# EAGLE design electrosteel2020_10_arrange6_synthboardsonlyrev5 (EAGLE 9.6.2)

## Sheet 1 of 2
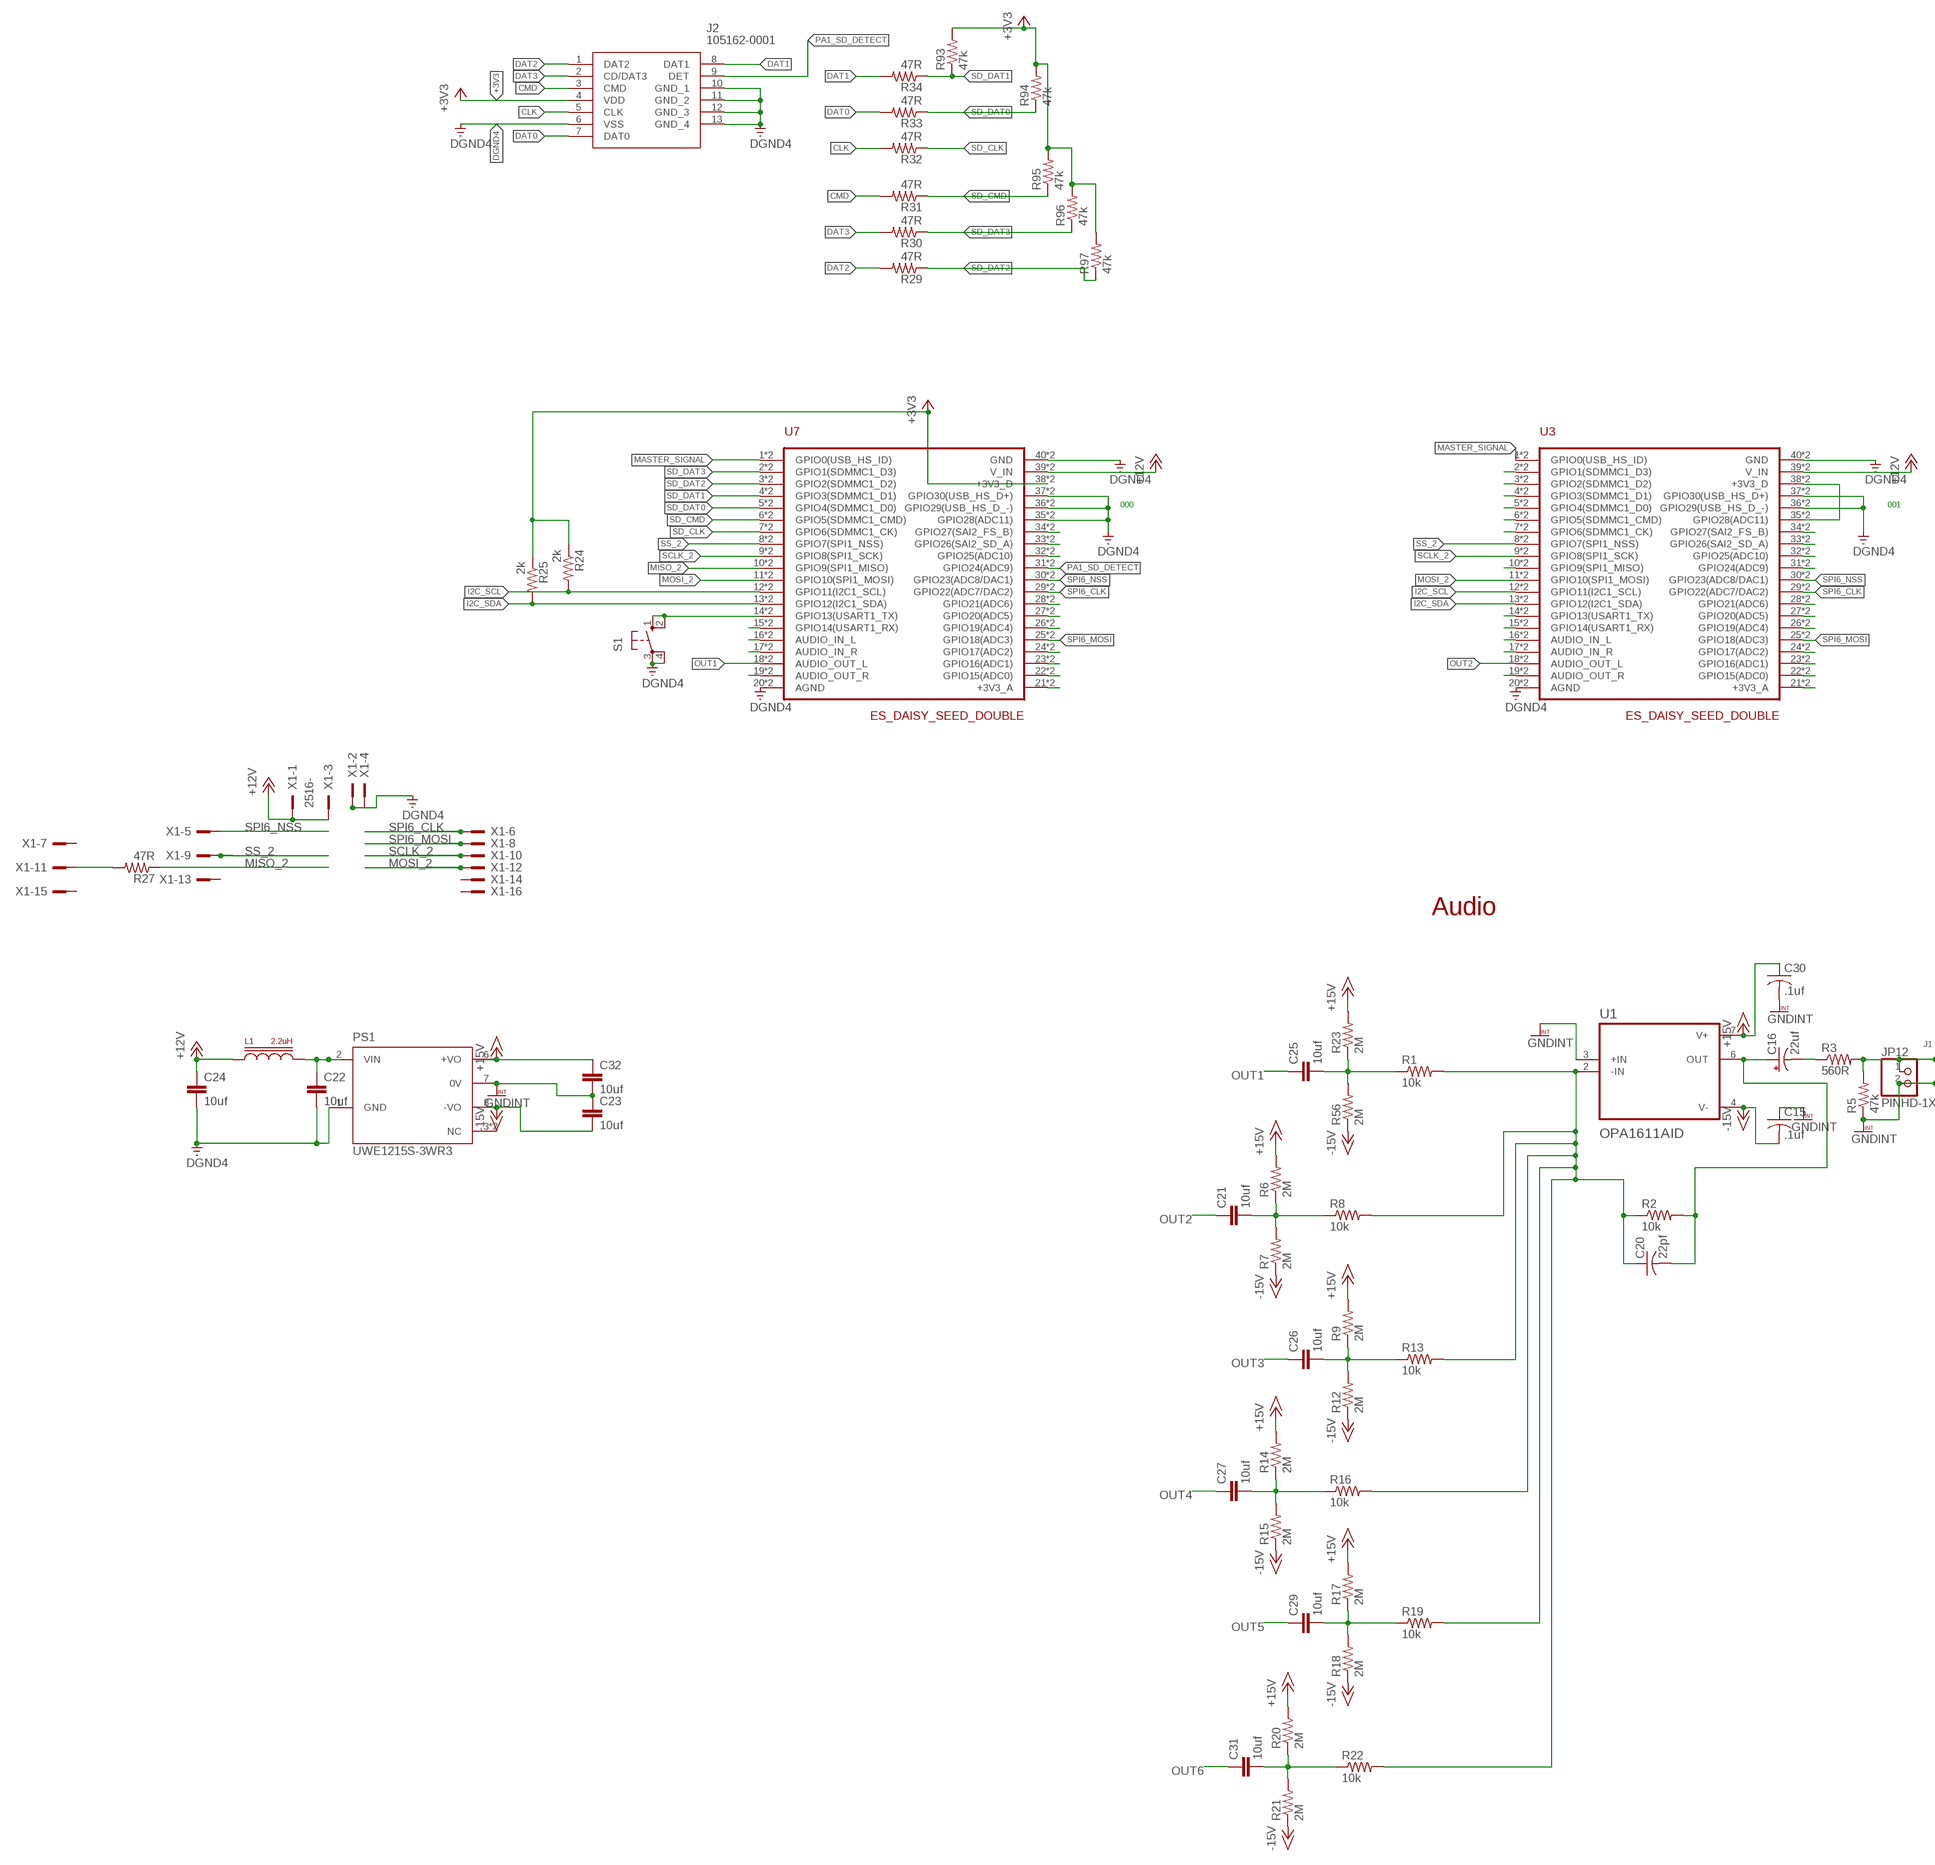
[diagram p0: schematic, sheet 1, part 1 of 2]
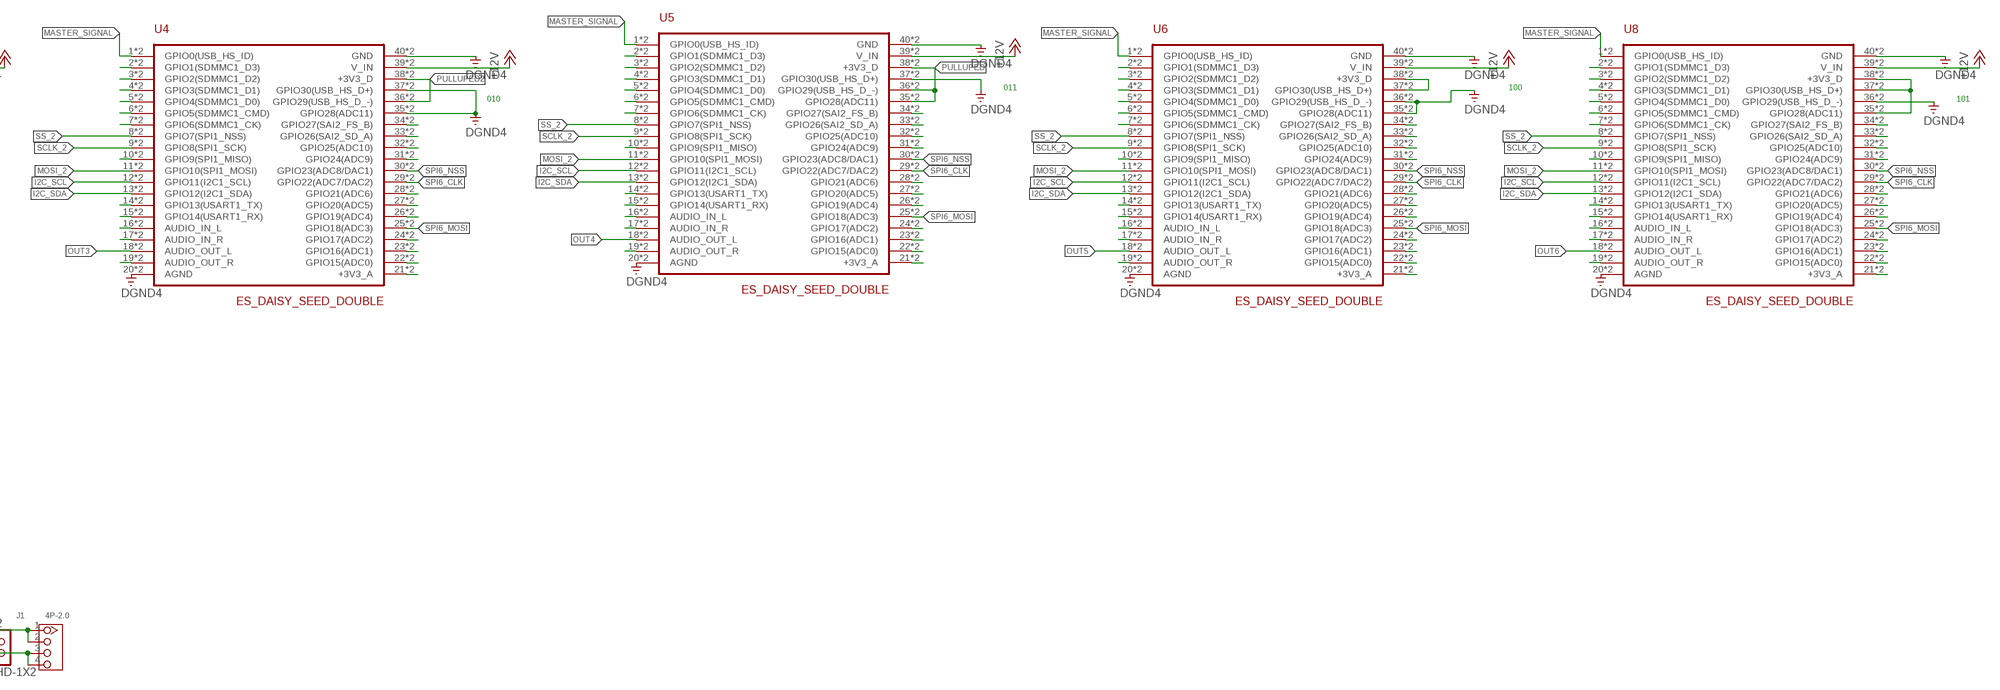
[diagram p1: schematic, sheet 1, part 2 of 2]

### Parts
C15  .1uf  C-USC0603K  [C0603K]
C16  22uf  CPOL-USD  [PANASONIC_D]
C20  22pf  C-USC0603  [C0603]
C21  10uf  C-EUC1206K  [C1206K]
C22  10uf  C-EUC1206K  [C1206K]
C23  10uf  C-EUC1206K  [C1206K]
C24  10uf  C-EUC1206K  [C1206K]
C25  10uf  C-EUC1206K  [C1206K]
C26  10uf  C-EUC1206K  [C1206K]
C27  10uf  C-EUC1206K  [C1206K]
C29  10uf  C-EUC1206K  [C1206K]
C30  .1uf  C-USC0603K  [C0603K]
C31  10uf  C-EUC1206K  [C1206K]
C32  10uf  C-EUC1206K  [C1206K]
J1  4P-2.0  GROVE-CONNECTOR-DIP(4P-2.0)  [HW4-2.0]
J2  105162-0001  [105162-0001]
JP12  PINHD-1X2  [1X02]
L1  2.2uH  INDUCTORS  [BOURNS_SRP2010]
PS1  UWE1215S-3WR3  [CONV_UWE1215S-3WR3]
R1  10k  R-US_R0603  [R0603]
R2  10k  R-US_R0603  [R0603]
R3  560R  R-US_R0603  [R0603]
R5  47k  R-US_R0603  [R0603]
R6  2M  R-US_R0603  [R0603]
R7  2M  R-US_R0603  [R0603]
R8  10k  R-US_R0603  [R0603]
R9  2M  R-US_R0603  [R0603]
R12  2M  R-US_R0603  [R0603]
R13  10k  R-US_R0603  [R0603]
R14  2M  R-US_R0603  [R0603]
R15  2M  R-US_R0603  [R0603]
R16  10k  R-US_R0603  [R0603]
R17  2M  R-US_R0603  [R0603]
R18  2M  R-US_R0603  [R0603]
R19  10k  R-US_R0603  [R0603]
R20  2M  R-US_R0603  [R0603]
R21  2M  R-US_R0603  [R0603]
R22  10k  R-US_R0603  [R0603]
R23  2M  R-US_R0603  [R0603]
R24  2k  R-US_R0603  [R0603]
R25  2k  R-US_R0603  [R0603]
R27  47R  R-US_R0603  [R0603]
R29  47R  R-US_R0603  [R0603]
R30  47R  R-US_R0603  [R0603]
R31  47R  R-US_R0603  [R0603]
R32  47R  R-US_R0603  [R0603]
R33  47R  R-US_R0603  [R0603]
R34  47R  R-US_R0603  [R0603]
R56  2M  R-US_R0603  [R0603]
R93  47k  R-US_R0603  [R0603]
R94  47k  R-US_R0603  [R0603]
R95  47k  R-US_R0603  [R0603]
R96  47k  R-US_R0603  [R0603]
R97  47k  R-US_R0603  [R0603]
S1  10-XX  [B3F-10XX]
U1  OPA1611AID  [SOIC127P599X175-8N]
U3  ES_DAISY_SEED_DOUBLE  [ES_DAISY_SEED_DOUBLE]
U4  ES_DAISY_SEED_DOUBLE  [ES_DAISY_SEED_DOUBLE]
U5  ES_DAISY_SEED_DOUBLE  [ES_DAISY_SEED_DOUBLE]
U6  ES_DAISY_SEED_DOUBLE  [ES_DAISY_SEED_DOUBLE]
U7  ES_DAISY_SEED_DOUBLE  [ES_DAISY_SEED_DOUBLE]
U8  ES_DAISY_SEED_DOUBLE  [ES_DAISY_SEED_DOUBLE]
X1  2516-  [PAK100/2500-16]

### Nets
+3V3: J2.4(VDD) R24.1 R25.1 R93.2 R94.2 R95.2 R96.2 R97.2 U7.38(+3V3_D) U7.B38(+3V3_D)
+12V: C24.1 L1.P$1 U3.39(V_IN) U3.B39(V_IN) U4.39(V_IN) U4.B39(V_IN) U5.39(V_IN) U5.B39(V_IN) U6.39(V_IN) U6.B39(V_IN) U7.39(V_IN) U7.B39(V_IN) U8.39(V_IN) U8.B39(V_IN) X1.1 X1.3
+15V: C30.1 C32.1 PS1.6(+VO) R6.2 R9.2 R14.2 R17.2 R20.2 R23.2 U1.7(V+)
-15V: C15.2 C23.2 PS1.8(-VO) R7.1 R12.1 R15.1 R18.1 R21.1 R56.1 U1.4(V-)
CLK: J2.5(CLK) R32.2
CMD: J2.3(CMD) R31.2
DAT0: J2.7(DAT0) R33.2
DAT1: J2.8(DAT1) R34.2
DAT2: J2.1(DAT2) R29.2
DAT3: J2.2(CD/DAT3) R30.2
DGND4: C22.2 C24.2 J2.6(VSS) J2.10(GND_1) J2.11(GND_2) J2.12(GND_3) J2.13(GND_4) PS1.1(GND) S1.3(P) S1.4(P1) U3.20(AGND) U3.36(GPIO29(USB_HS_D_-)) U3.37(GPIO30(USB_HS_D+)) U3.40(GND) U3.B20(AGND) U3.B36(GPIO29(USB_HS_D_-)) U3.B37(GPIO30(USB_HS_D+)) U3.B40(GND) U4.20(AGND) U4.35(GPIO28(ADC11)) U4.37(GPIO30(USB_HS_D+)) U4.40(GND) U4.B20(AGND) U4.B35(GPIO28(ADC11)) U4.B37(GPIO30(USB_HS_D+)) U4.B40(GND) U5.20(AGND) U5.37(GPIO30(USB_HS_D+)) U5.40(GND) U5.B20(AGND) U5.B37(GPIO30(USB_HS_D+)) U5.B40(GND) U6.20(AGND) U6.35(GPIO28(ADC11)) U6.36(GPIO29(USB_HS_D_-)) U6.40(GND) U6.B20(AGND) U6.B35(GPIO28(ADC11)) U6.B36(GPIO29(USB_HS_D_-)) U6.B40(GND) U7.20(AGND) U7.35(GPIO28(ADC11)) U7.36(GPIO29(USB_HS_D_-)) U7.37(GPIO30(USB_HS_D+)) U7.40(GND) U7.B20(AGND) U7.B35(GPIO28(ADC11)) U7.B36(GPIO29(USB_HS_D_-)) U7.B37(GPIO30(USB_HS_D+)) U7.B40(GND) U8.20(AGND) U8.36(GPIO29(USB_HS_D_-)) U8.40(GND) U8.B20(AGND) U8.B36(GPIO29(USB_HS_D_-)) U8.B40(GND) X1.2 X1.4
GNDINT: C15.1 C23.1 C30.2 C32.2 J1.3 J1.4 JP12.2 PS1.7(0V) R5.1 U1.3(+IN)
I2C_SCL: R24.2 U3.12(GPIO11(I2C1_SCL)) U3.B12(GPIO11(I2C1_SCL)) U4.12(GPIO11(I2C1_SCL)) U4.B12(GPIO11(I2C1_SCL)) U5.12(GPIO11(I2C1_SCL)) U5.B12(GPIO11(I2C1_SCL)) U6.12(GPIO11(I2C1_SCL)) U6.B12(GPIO11(I2C1_SCL)) U7.12(GPIO11(I2C1_SCL)) U7.B12(GPIO11(I2C1_SCL)) U8.12(GPIO11(I2C1_SCL)) U8.B12(GPIO11(I2C1_SCL))
I2C_SDA: R25.2 U3.13(GPIO12(I2C1_SDA)) U3.B13(GPIO12(I2C1_SDA)) U4.13(GPIO12(I2C1_SDA)) U4.B13(GPIO12(I2C1_SDA)) U5.13(GPIO12(I2C1_SDA)) U5.B13(GPIO12(I2C1_SDA)) U6.13(GPIO12(I2C1_SDA)) U6.B13(GPIO12(I2C1_SDA)) U7.13(GPIO12(I2C1_SDA)) U7.B13(GPIO12(I2C1_SDA)) U8.13(GPIO12(I2C1_SDA)) U8.B13(GPIO12(I2C1_SDA))
MASTER_SIGNAL: U3.1(GPIO0(USB_HS_ID)) U3.B1(GPIO0(USB_HS_ID)) U4.1(GPIO0(USB_HS_ID)) U4.B1(GPIO0(USB_HS_ID)) U5.1(GPIO0(USB_HS_ID)) U5.B1(GPIO0(USB_HS_ID)) U6.1(GPIO0(USB_HS_ID)) U6.B1(GPIO0(USB_HS_ID)) U7.1(GPIO0(USB_HS_ID)) U7.B1(GPIO0(USB_HS_ID)) U8.1(GPIO0(USB_HS_ID)) U8.B1(GPIO0(USB_HS_ID))
MISO_2: R27.1 U7.10(GPIO9(SPI1_MISO)) U7.B10(GPIO9(SPI1_MISO))
MISO_2_P1: U3.10(GPIO9(SPI1_MISO)) U3.B10(GPIO9(SPI1_MISO))
MISO_2_P2: U4.10(GPIO9(SPI1_MISO)) U4.B10(GPIO9(SPI1_MISO))
MISO_2_P3: U5.10(GPIO9(SPI1_MISO)) U5.B10(GPIO9(SPI1_MISO))
MISO_2_P4: U6.10(GPIO9(SPI1_MISO)) U6.B10(GPIO9(SPI1_MISO))
MISO_2_P5: U8.10(GPIO9(SPI1_MISO)) U8.B10(GPIO9(SPI1_MISO))
MONO_OUTPUT: C16.+ C20.2 R2.2 U1.6(OUT)
MOSI_2: U3.11(GPIO10(SPI1_MOSI)) U3.B11(GPIO10(SPI1_MOSI)) U4.11(GPIO10(SPI1_MOSI)) U4.B11(GPIO10(SPI1_MOSI)) U5.11(GPIO10(SPI1_MOSI)) U5.B11(GPIO10(SPI1_MOSI)) U6.11(GPIO10(SPI1_MOSI)) U6.B11(GPIO10(SPI1_MOSI)) U7.11(GPIO10(SPI1_MOSI)) U7.B11(GPIO10(SPI1_MOSI)) U8.11(GPIO10(SPI1_MOSI)) U8.B11(GPIO10(SPI1_MOSI)) X1.12
N$1: U5.31(GPIO24(ADC9)) U5.B31(GPIO24(ADC9))
N$2: C21.2 R6.1 R7.2 R8.1
N$3: U6.31(GPIO24(ADC9)) U6.B31(GPIO24(ADC9))
N$4: C20.1 R1.2 R2.1 R8.2 R13.2 R16.2 R19.2 R22.2 U1.2(-IN)
N$5: C16.- R3.1
N$6: J1.1 J1.2 JP12.1 R3.2 R5.2
N$7: C25.2 R1.1 R23.1 R56.2
N$8: C26.2 R9.1 R12.2 R13.1
N$9: C27.2 R14.1 R15.2 R16.1
N$10: C29.2 R17.1 R18.2 R19.1
N$11: C31.2 R20.1 R21.2 R22.1
N$12: U7.19(AUDIO_OUT_R) U7.B19(AUDIO_OUT_R)
N$13: U7.17(AUDIO_IN_R) U7.B17(AUDIO_IN_R)
N$14: U7.16(AUDIO_IN_L) U7.B16(AUDIO_IN_L)
N$15: U7.15(GPIO14(USART1_RX)) U7.B15(GPIO14(USART1_RX))
N$17: U8.31(GPIO24(ADC9)) U8.B31(GPIO24(ADC9))
N$18: U8.26(GPIO19(ADC4)) U8.B26(GPIO19(ADC4))
N$19: U6.26(GPIO19(ADC4)) U6.B26(GPIO19(ADC4))
N$20: U7.34(GPIO27(SAI2_FS_B)) U7.B34(GPIO27(SAI2_FS_B))
N$21: U7.33(GPIO26(SAI2_SD_A)) U7.B33(GPIO26(SAI2_SD_A))
N$22: U7.32(GPIO25(ADC10)) U7.B32(GPIO25(ADC10))
N$23: U5.26(GPIO19(ADC4)) U5.B26(GPIO19(ADC4))
N$24: R27.2 X1.11
N$25: U7.28(GPIO21(ADC6)) U7.B28(GPIO21(ADC6))
N$26: U7.27(GPIO20(ADC5)) U7.B27(GPIO20(ADC5))
N$27: U4.26(GPIO19(ADC4)) U4.B26(GPIO19(ADC4))
N$28: U3.26(GPIO19(ADC4)) U3.B26(GPIO19(ADC4))
N$29: U3.21(+3V3_A) U3.B21(+3V3_A)
N$30: U7.24(GPIO17(ADC2)) U7.B24(GPIO17(ADC2))
N$31: U7.23(GPIO16(ADC1)) U7.B23(GPIO16(ADC1))
N$32: U7.22(GPIO15(ADC0)) U7.B22(GPIO15(ADC0))
N$33: U3.19(AUDIO_OUT_R) U3.B19(AUDIO_OUT_R)
N$34: U3.17(AUDIO_IN_R) U3.B17(AUDIO_IN_R)
N$35: U3.16(AUDIO_IN_L) U3.B16(AUDIO_IN_L)
N$36: U3.15(GPIO14(USART1_RX)) U3.B15(GPIO14(USART1_RX))
N$37: U3.14(GPIO13(USART1_TX)) U3.B14(GPIO13(USART1_TX))
N$38: U7.26(GPIO19(ADC4)) U7.B26(GPIO19(ADC4))
N$39: U3.35(GPIO28(ADC11)) U3.38(+3V3_D) U3.B35(GPIO28(ADC11)) U3.B38(+3V3_D)
N$40: U3.34(GPIO27(SAI2_FS_B)) U3.B34(GPIO27(SAI2_FS_B))
N$41: U3.33(GPIO26(SAI2_SD_A)) U3.B33(GPIO26(SAI2_SD_A))
N$42: U3.32(GPIO25(ADC10)) U3.B32(GPIO25(ADC10))
N$43: U3.28(GPIO21(ADC6)) U3.B28(GPIO21(ADC6))
N$44: U3.27(GPIO20(ADC5)) U3.B27(GPIO20(ADC5))
N$45: U7.21(+3V3_A) U7.B21(+3V3_A)
N$46: U3.24(GPIO17(ADC2)) U3.B24(GPIO17(ADC2))
N$47: U3.23(GPIO16(ADC1)) U3.B23(GPIO16(ADC1))
N$48: U3.22(GPIO15(ADC0)) U3.B22(GPIO15(ADC0))
N$49: U4.21(+3V3_A) U4.B21(+3V3_A)
N$50: U4.19(AUDIO_OUT_R) U4.B19(AUDIO_OUT_R)
N$51: U4.17(AUDIO_IN_R) U4.B17(AUDIO_IN_R)
N$52: U4.16(AUDIO_IN_L) U4.B16(AUDIO_IN_L)
N$53: U4.15(GPIO14(USART1_RX)) U4.B15(GPIO14(USART1_RX))
N$54: U4.14(GPIO13(USART1_TX)) U4.B14(GPIO13(USART1_TX))
N$55: S1.1(S) S1.2(S1) U7.14(GPIO13(USART1_TX)) U7.B14(GPIO13(USART1_TX))
N$56: U3.2(GPIO1(SDMMC1_D3)) U3.B2(GPIO1(SDMMC1_D3))
N$57: U4.34(GPIO27(SAI2_FS_B)) U4.B34(GPIO27(SAI2_FS_B))
N$58: U4.33(GPIO26(SAI2_SD_A)) U4.B33(GPIO26(SAI2_SD_A))
N$59: U4.32(GPIO25(ADC10)) U4.B32(GPIO25(ADC10))
N$60: U4.28(GPIO21(ADC6)) U4.B28(GPIO21(ADC6))
N$61: U4.27(GPIO20(ADC5)) U4.B27(GPIO20(ADC5))
N$62: U4.24(GPIO17(ADC2)) U4.B24(GPIO17(ADC2))
N$63: U4.23(GPIO16(ADC1)) U4.B23(GPIO16(ADC1))
N$64: U4.22(GPIO15(ADC0)) U4.B22(GPIO15(ADC0))
N$65: U5.21(+3V3_A) U5.B21(+3V3_A)
N$66: U5.19(AUDIO_OUT_R) U5.B19(AUDIO_OUT_R)
N$67: U5.17(AUDIO_IN_R) U5.B17(AUDIO_IN_R)
N$68: U5.16(AUDIO_IN_L) U5.B16(AUDIO_IN_L)
N$69: U5.15(GPIO14(USART1_RX)) U5.B15(GPIO14(USART1_RX))
N$70: U5.14(GPIO13(USART1_TX)) U5.B14(GPIO13(USART1_TX))
N$71: U3.3(GPIO2(SDMMC1_D2)) U3.B3(GPIO2(SDMMC1_D2))
N$72: U3.4(GPIO3(SDMMC1_D1)) U3.B4(GPIO3(SDMMC1_D1))
N$73: U5.34(GPIO27(SAI2_FS_B)) U5.B34(GPIO27(SAI2_FS_B))
N$74: U5.33(GPIO26(SAI2_SD_A)) U5.B33(GPIO26(SAI2_SD_A))
N$75: U5.32(GPIO25(ADC10)) U5.B32(GPIO25(ADC10))
N$76: U5.28(GPIO21(ADC6)) U5.B28(GPIO21(ADC6))
N$77: U5.27(GPIO20(ADC5)) U5.B27(GPIO20(ADC5))
N$78: U5.24(GPIO17(ADC2)) U5.B24(GPIO17(ADC2))
N$79: U5.23(GPIO16(ADC1)) U5.B23(GPIO16(ADC1))
N$80: U5.22(GPIO15(ADC0)) U5.B22(GPIO15(ADC0))
N$81: C22.1 L1.P$2 PS1.2(VIN)
N$82: U6.21(+3V3_A) U6.B21(+3V3_A)
N$83: U6.19(AUDIO_OUT_R) U6.B19(AUDIO_OUT_R)
N$84: U6.17(AUDIO_IN_R) U6.B17(AUDIO_IN_R)
N$85: U6.16(AUDIO_IN_L) U6.B16(AUDIO_IN_L)
N$86: U6.15(GPIO14(USART1_RX)) U6.B15(GPIO14(USART1_RX))
N$87: U6.14(GPIO13(USART1_TX)) U6.B14(GPIO13(USART1_TX))
N$88: U6.37(GPIO30(USB_HS_D+)) U6.38(+3V3_D) U6.B37(GPIO30(USB_HS_D+)) U6.B38(+3V3_D)
N$89: U3.5(GPIO4(SDMMC1_D0)) U3.B5(GPIO4(SDMMC1_D0))
N$90: U6.34(GPIO27(SAI2_FS_B)) U6.B34(GPIO27(SAI2_FS_B))
N$91: U6.33(GPIO26(SAI2_SD_A)) U6.B33(GPIO26(SAI2_SD_A))
N$92: U6.32(GPIO25(ADC10)) U6.B32(GPIO25(ADC10))
N$93: U6.28(GPIO21(ADC6)) U6.B28(GPIO21(ADC6))
N$94: U6.27(GPIO20(ADC5)) U6.B27(GPIO20(ADC5))
N$95: U6.24(GPIO17(ADC2)) U6.B24(GPIO17(ADC2))
N$96: U6.23(GPIO16(ADC1)) U6.B23(GPIO16(ADC1))
N$97: U6.22(GPIO15(ADC0)) U6.B22(GPIO15(ADC0))
N$98: U8.21(+3V3_A) U8.B21(+3V3_A)
N$99: U8.19(AUDIO_OUT_R) U8.B19(AUDIO_OUT_R)
N$100: U8.17(AUDIO_IN_R) U8.B17(AUDIO_IN_R)
N$101: U8.16(AUDIO_IN_L) U8.B16(AUDIO_IN_L)
N$102: U8.15(GPIO14(USART1_RX)) U8.B15(GPIO14(USART1_RX))
N$103: U8.14(GPIO13(USART1_TX)) U8.B14(GPIO13(USART1_TX))
N$104: U8.35(GPIO28(ADC11)) U8.37(GPIO30(USB_HS_D+)) U8.38(+3V3_D) U8.B35(GPIO28(ADC11)) U8.B37(GPIO30(USB_HS_D+)) U8.B38(+3V3_D)
N$105: U3.6(GPIO5(SDMMC1_CMD)) U3.B6(GPIO5(SDMMC1_CMD))
N$106: U3.7(GPIO6(SDMMC1_CK)) U3.B7(GPIO6(SDMMC1_CK))
N$108: U8.34(GPIO27(SAI2_FS_B)) U8.B34(GPIO27(SAI2_FS_B))
N$109: U8.33(GPIO26(SAI2_SD_A)) U8.B33(GPIO26(SAI2_SD_A))
N$110: U8.32(GPIO25(ADC10)) U8.B32(GPIO25(ADC10))
N$111: U8.28(GPIO21(ADC6)) U8.B28(GPIO21(ADC6))
N$112: U8.27(GPIO20(ADC5)) U8.B27(GPIO20(ADC5))
N$113: U8.24(GPIO17(ADC2)) U8.B24(GPIO17(ADC2))
N$114: U8.23(GPIO16(ADC1)) U8.B23(GPIO16(ADC1))
N$115: U8.22(GPIO15(ADC0)) U8.B22(GPIO15(ADC0))
N$116: U4.2(GPIO1(SDMMC1_D3)) U4.B2(GPIO1(SDMMC1_D3))
N$117: U4.3(GPIO2(SDMMC1_D2)) U4.B3(GPIO2(SDMMC1_D2))
N$118: U4.4(GPIO3(SDMMC1_D1)) U4.B4(GPIO3(SDMMC1_D1))
N$119: U4.5(GPIO4(SDMMC1_D0)) U4.B5(GPIO4(SDMMC1_D0))
N$120: U4.6(GPIO5(SDMMC1_CMD)) U4.B6(GPIO5(SDMMC1_CMD))
N$121: U4.7(GPIO6(SDMMC1_CK)) U4.B7(GPIO6(SDMMC1_CK))
N$123: U5.2(GPIO1(SDMMC1_D3)) U5.B2(GPIO1(SDMMC1_D3))
N$124: U5.3(GPIO2(SDMMC1_D2)) U5.B3(GPIO2(SDMMC1_D2))
N$125: U5.4(GPIO3(SDMMC1_D1)) U5.B4(GPIO3(SDMMC1_D1))
N$126: U5.5(GPIO4(SDMMC1_D0)) U5.B5(GPIO4(SDMMC1_D0))
N$127: U5.6(GPIO5(SDMMC1_CMD)) U5.B6(GPIO5(SDMMC1_CMD))
N$128: U5.7(GPIO6(SDMMC1_CK)) U5.B7(GPIO6(SDMMC1_CK))
N$130: U6.2(GPIO1(SDMMC1_D3)) U6.B2(GPIO1(SDMMC1_D3))
N$131: U6.3(GPIO2(SDMMC1_D2)) U6.B3(GPIO2(SDMMC1_D2))
N$132: U6.4(GPIO3(SDMMC1_D1)) U6.B4(GPIO3(SDMMC1_D1))
N$133: U6.5(GPIO4(SDMMC1_D0)) U6.B5(GPIO4(SDMMC1_D0))
N$134: U6.6(GPIO5(SDMMC1_CMD)) U6.B6(GPIO5(SDMMC1_CMD))
N$135: U6.7(GPIO6(SDMMC1_CK)) U6.B7(GPIO6(SDMMC1_CK))
N$136: U8.2(GPIO1(SDMMC1_D3)) U8.B2(GPIO1(SDMMC1_D3))
N$137: U8.3(GPIO2(SDMMC1_D2)) U8.B3(GPIO2(SDMMC1_D2))
N$138: U8.4(GPIO3(SDMMC1_D1)) U8.B4(GPIO3(SDMMC1_D1))
N$139: U8.5(GPIO4(SDMMC1_D0)) U8.B5(GPIO4(SDMMC1_D0))
N$140: U8.6(GPIO5(SDMMC1_CMD)) U8.B6(GPIO5(SDMMC1_CMD))
N$141: U8.7(GPIO6(SDMMC1_CK)) U8.B7(GPIO6(SDMMC1_CK))
OUT1: C25.1 U7.18(AUDIO_OUT_L) U7.B18(AUDIO_OUT_L)
OUT2: C21.1 U3.18(AUDIO_OUT_L) U3.B18(AUDIO_OUT_L)
OUT3: C26.1 U4.18(AUDIO_OUT_L) U4.B18(AUDIO_OUT_L)
OUT4: C27.1 U5.18(AUDIO_OUT_L) U5.B18(AUDIO_OUT_L)
OUT5: C29.1 U6.18(AUDIO_OUT_L) U6.B18(AUDIO_OUT_L)
OUT6: C31.1 U8.18(AUDIO_OUT_L) U8.B18(AUDIO_OUT_L)
PA1_SD_DETECT: J2.9(DET) U3.31(GPIO24(ADC9)) U3.B31(GPIO24(ADC9)) U7.31(GPIO24(ADC9)) U7.B31(GPIO24(ADC9))
PA1_SD_DETECT1: U4.31(GPIO24(ADC9)) U4.B31(GPIO24(ADC9))
PULLUPED: U5.35(GPIO28(ADC11)) U5.36(GPIO29(USB_HS_D_-)) U5.38(+3V3_D) U5.B35(GPIO28(ADC11)) U5.B36(GPIO29(USB_HS_D_-)) U5.B38(+3V3_D)
PULLUPED2: U4.36(GPIO29(USB_HS_D_-)) U4.38(+3V3_D) U4.B36(GPIO29(USB_HS_D_-)) U4.B38(+3V3_D)
SCLK_2: U3.9(GPIO8(SPI1_SCK)) U3.B9(GPIO8(SPI1_SCK)) U4.9(GPIO8(SPI1_SCK)) U4.B9(GPIO8(SPI1_SCK)) U5.9(GPIO8(SPI1_SCK)) U5.B9(GPIO8(SPI1_SCK)) U6.9(GPIO8(SPI1_SCK)) U6.B9(GPIO8(SPI1_SCK)) U7.9(GPIO8(SPI1_SCK)) U7.B9(GPIO8(SPI1_SCK)) U8.9(GPIO8(SPI1_SCK)) U8.B9(GPIO8(SPI1_SCK)) X1.10
SD_CLK: R32.1 U7.7(GPIO6(SDMMC1_CK)) U7.B7(GPIO6(SDMMC1_CK))
SD_CMD: R31.1 R95.1 U7.6(GPIO5(SDMMC1_CMD)) U7.B6(GPIO5(SDMMC1_CMD))
SD_DAT0: R33.1 R94.1 U7.5(GPIO4(SDMMC1_D0)) U7.B5(GPIO4(SDMMC1_D0))
SD_DAT1: R34.1 R93.1 U7.4(GPIO3(SDMMC1_D1)) U7.B4(GPIO3(SDMMC1_D1))
SD_DAT2: R29.1 R97.1 U7.3(GPIO2(SDMMC1_D2)) U7.B3(GPIO2(SDMMC1_D2))
SD_DAT3: R30.1 R96.1 U7.2(GPIO1(SDMMC1_D3)) U7.B2(GPIO1(SDMMC1_D3))
SPI6_CLK: U3.29(GPIO22(ADC7/DAC2)) U3.B29(GPIO22(ADC7/DAC2)) U4.29(GPIO22(ADC7/DAC2)) U4.B29(GPIO22(ADC7/DAC2)) U5.29(GPIO22(ADC7/DAC2)) U5.B29(GPIO22(ADC7/DAC2)) U6.29(GPIO22(ADC7/DAC2)) U6.B29(GPIO22(ADC7/DAC2)) U7.29(GPIO22(ADC7/DAC2)) U7.B29(GPIO22(ADC7/DAC2)) U8.29(GPIO22(ADC7/DAC2)) U8.B29(GPIO22(ADC7/DAC2)) X1.6
SPI6_MOSI: U3.25(GPIO18(ADC3)) U3.B25(GPIO18(ADC3)) U4.25(GPIO18(ADC3)) U4.B25(GPIO18(ADC3)) U5.25(GPIO18(ADC3)) U5.B25(GPIO18(ADC3)) U6.25(GPIO18(ADC3)) U6.B25(GPIO18(ADC3)) U7.25(GPIO18(ADC3)) U7.B25(GPIO18(ADC3)) U8.25(GPIO18(ADC3)) U8.B25(GPIO18(ADC3)) X1.8
SPI6_NSS: U3.30(GPIO23(ADC8/DAC1)) U3.B30(GPIO23(ADC8/DAC1)) U4.30(GPIO23(ADC8/DAC1)) U4.B30(GPIO23(ADC8/DAC1)) U5.30(GPIO23(ADC8/DAC1)) U5.B30(GPIO23(ADC8/DAC1)) U6.30(GPIO23(ADC8/DAC1)) U6.B30(GPIO23(ADC8/DAC1)) U7.30(GPIO23(ADC8/DAC1)) U7.B30(GPIO23(ADC8/DAC1)) U8.30(GPIO23(ADC8/DAC1)) U8.B30(GPIO23(ADC8/DAC1)) X1.5
SS_2: U3.8(GPIO7(SPI1_NSS)) U3.B8(GPIO7(SPI1_NSS)) U4.8(GPIO7(SPI1_NSS)) U4.B8(GPIO7(SPI1_NSS)) U5.8(GPIO7(SPI1_NSS)) U5.B8(GPIO7(SPI1_NSS)) U6.8(GPIO7(SPI1_NSS)) U6.B8(GPIO7(SPI1_NSS)) U7.8(GPIO7(SPI1_NSS)) U7.B8(GPIO7(SPI1_NSS)) U8.8(GPIO7(SPI1_NSS)) U8.B8(GPIO7(SPI1_NSS)) X1.9
Unconnected: PS1.3(NC) PS1.5(NC) X1.7 X1.13 X1.14 X1.15 X1.16

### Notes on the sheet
- 011 | 100
- 000 | 001 | 010 | 101
- Audio

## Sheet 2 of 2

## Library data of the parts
C15 C30 = rcl:C-US: CAPACITOR, American symbol; PARTNO: CC0603KRX7R8BB104
C16 = adafruit:CPOL-US: POLARIZED CAPACITOR, American symbol; PARTNO: EEE-1CA220NP
C20 = rcl:C-US: CAPACITOR, American symbol; PARTNO: CC0603JRNPO9BN220; SPICEPREFIX: C
C21-C27 C29 C31 C32 = rcl:C-EU: CAPACITOR, European symbol; PARTNO: TMK316F106ZL-T
J1 = OPL_Connector:GROVE-CONNECTOR-DIP(4P-2.0): 320110033; PARTNO: 110990030
J2 = 105162-0001:105162-0001: Memory Card Connectors 1.45H MICRO SD HEADER WITH D/C PIN Source: Datasheet Check prices; AVAILABILITY: In Stock; DESCRIPTION: 9 (8 + 1) Position Card Connector Secure Digital - microSD™ Surface Mount, Right Angle Gold; MF: Molex; MP: 1051620001; PACKAGE: None; PARTNO: 105162-0001; PRICE: None; PURCHASE-URL: https://pricing.snapeda.com/search/part/1051620001/?ref=eda
JP12 = Connector:PINHD-1X2: PIN HEADER; CATEGORY: CONNECTOR; PARTNO: *DNP; SUB-CATEGORY: PIN-HEADER
L1 = Electrosmith-Passives:INDUCTOR; PARTNO: SRP2010-2R2M
PS1 = UWE1215S-3WR3:UWE1215S-3WR3: DC/DC Converter; DESCRIPTION: Isolated Module DC DC Converter 2 Output 15V -15V - - 100mA, 100mA 4.5V - 36V Input; DIGI-KEY_PART_NUMBER: 2725-UWE1215S-3WR3-ND; MF: Mornsun America, LLC; MP: UWE1215S-3WR3; PACKAGE: SIP-7-7 MORNSUN; PARTNO: UWE1215S-3WR3; PURCHASE-URL: https://pricing.snapeda.com/search/part/UWE1215S-3WR3/?ref=eda
R1 R2 R8 R13 R16 R19 R22 = Resistor:R-US_: RESISTOR, American symbol; PARTNO: ESR03EZPF1002
R3 = Resistor:R-US_: RESISTOR, American symbol; PARTNO: ESR03EZPF5600
R5 = Resistor:R-US_: RESISTOR, American symbol; PARTNO: ESR03EZPJ473
R6 R7 R9 R12 R14 R15 R17 R18 R20 R21 R23 R56 = Electrosmith-Passives:R-US_: RESISTOR, American symbol; PACKAGE: R0603; PARTNO: RMCF0603FT2M00
R24 R25 = rcl:R-US_: RESISTOR, American symbol; PARTNO: ERJ-PA3F2001V; SPICEPREFIX: R
R27 R29-R34 = rcl:R-US_: RESISTOR, American symbol; PARTNO: RC0603JR-0747RL; SPICEPREFIX: R
R93-R97 = rcl:R-US_: RESISTOR, American symbol; PARTNO: ESR03EZPJ473
S1 = switch-omron:10-XX: OMRON SWITCH; MPN: B3F-1000; OC_FARNELL: 176432; OC_NEWARK: 36M3542
U1 = OPA1611AID:OPA1611AID; DESCRIPTION: 1.1nV/√Hz Noise, Low Power, Precision Operational Amplifier; DIGI-KEY_PART_NUMBER: 296-24958-5-ND; MF: Texas Instruments; MP: OPA1611AID; PACKAGE: SOIC-8 Texas Instruments; PARTNO: OPA1611AID; PURCHASE-URL: https://pricing.snapeda.com/search/part/OPA1611AID/?ref=eda
U3-U8 = Electrosmith_Boards:ES_DAISY_SEED; PARTNO: 4840-6004-CP
X1 = con-3m:2516-: 3M (TM) Pak 100 4-Wall Header Source: 3M; OC_FARNELL: unknown; OC_NEWARK: unknown; PARTNO: SBH11-PBPC-D08-ST-BK

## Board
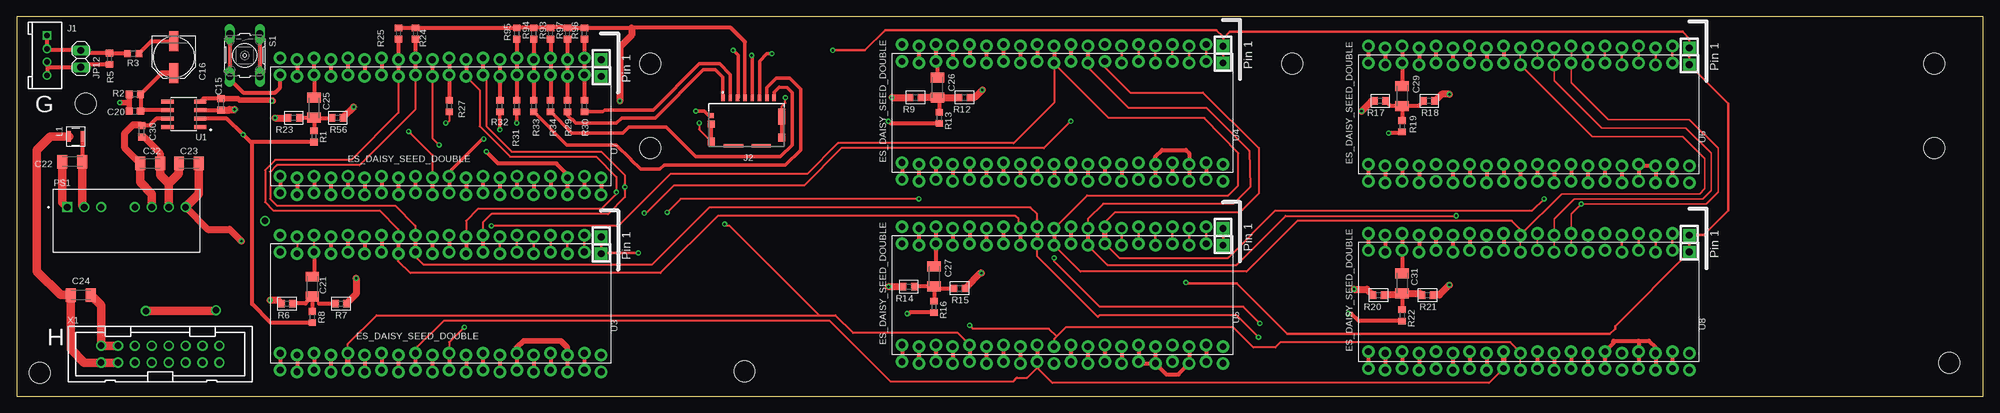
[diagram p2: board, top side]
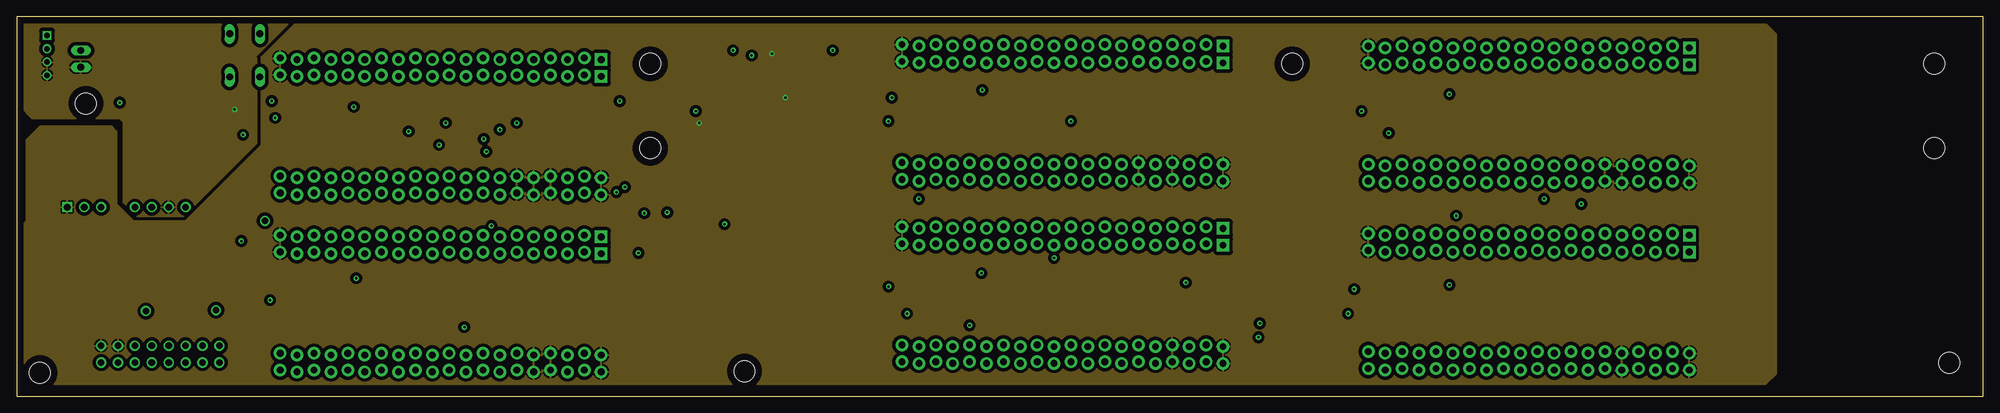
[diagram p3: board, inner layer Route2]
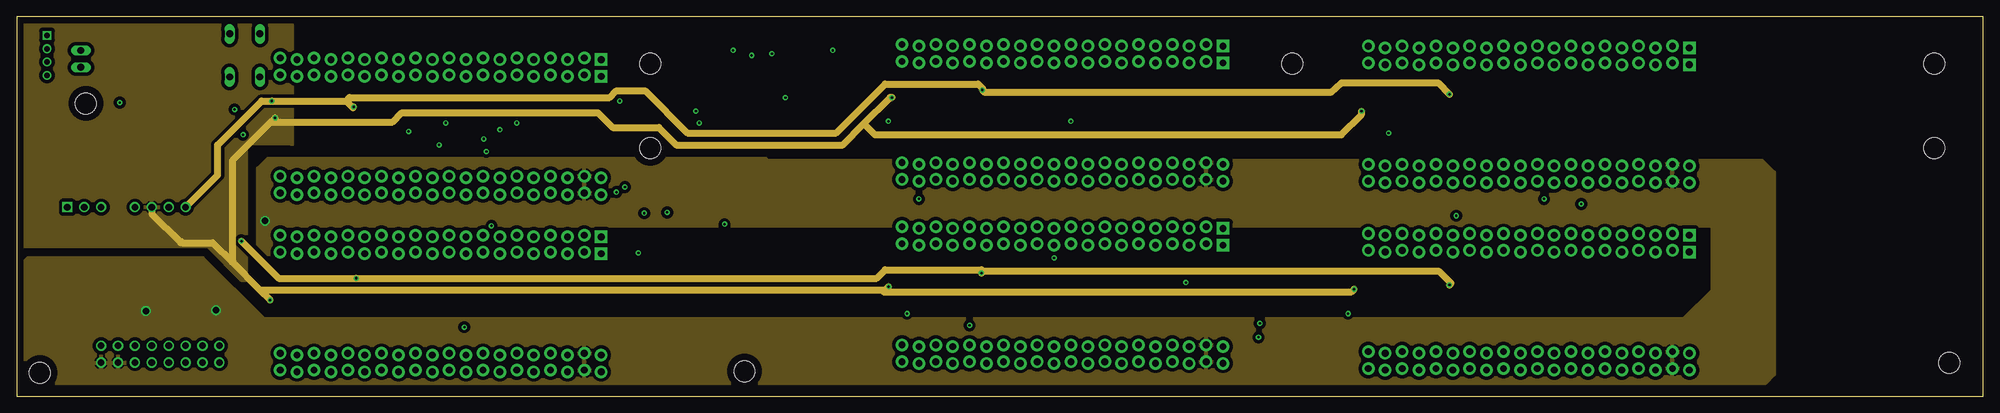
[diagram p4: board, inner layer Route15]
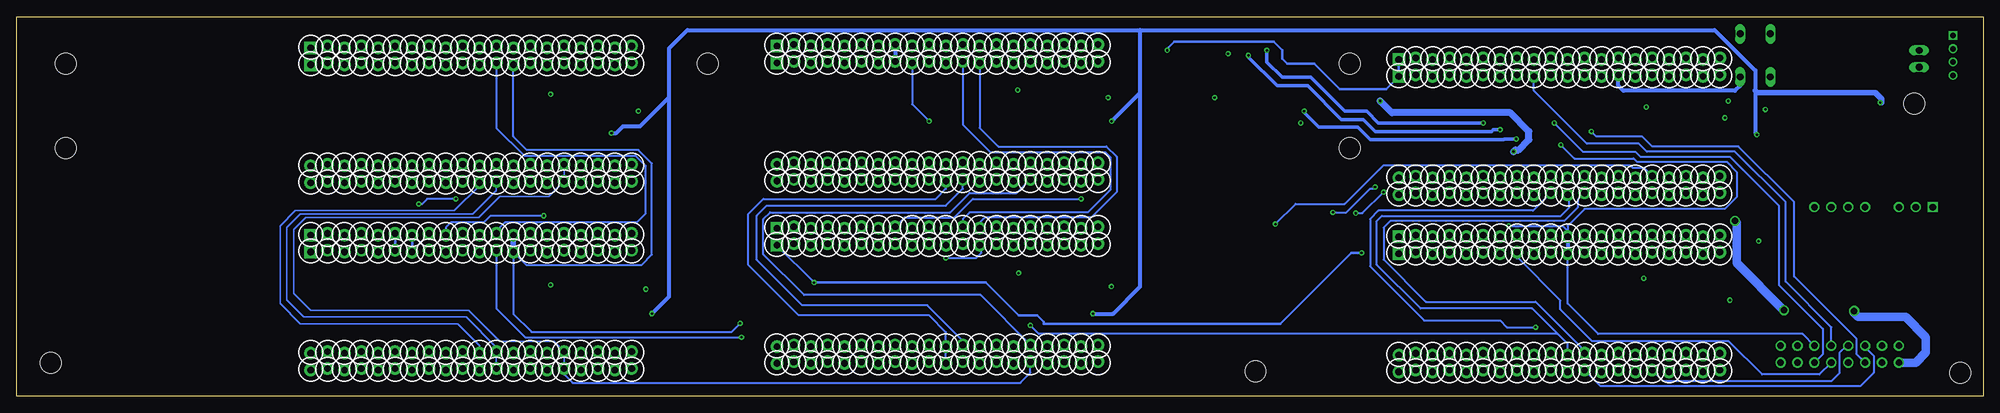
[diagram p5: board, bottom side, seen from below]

Size 295.66 x 57.15 mm. Coordinates in mm from the lower left corner, seen from the top.
Outline: 0,57.15 0,0 295.66,0 295.66,57.15 0,57.15
Copper layers (1+2*15+16): Top 0.035mm / dielectric 0.5mm / Route2 0.035mm / dielectric 0.5mm / Route15 0.035mm / dielectric 0.5mm / Bottom 0.035mm
Design rules "default *": minimum track width 6mil, minimum drill 0.35mm, track to track 9mil, track to pad 9mil, pad to pad 9mil, via to via 9mil, smd to smd 9mil, copper to edge 40mil, drill to drill 6mil, minimum pad ring 10mil, minimum via ring 8mil, stop-mask expansion 4mil, vias tented up to drill 0mil, thermal gap 10mil
Holes 3.17 mm at 95.25,37.34 288.29,37.34 10.41,44.07 290.53,5.05 109.42,3.78 3.51,3.53 288.29,50.04 191.77,50.04 95.25,50.04

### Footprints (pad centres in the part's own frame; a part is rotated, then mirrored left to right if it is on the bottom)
C0603K = smd 1.05 x 1.08: 1 -0.875,0; 2 0.875,0
PANASONIC_D = smd 3 x 1.4: + 2.4,0; - -2.4,0
C0603 = smd 1.1 x 1: 1 -0.85,0; 2 0.85,0
C1206K = smd 1.5 x 2: 1 -1.5,0; 2 1.5,0
HW4-2.0 = drill 0.8 pad 1.27 square: 1 -3,0 | drill 0.8 pad 1.27: 2 -1,0; 3 1,0; 4 3,0
105162-0001 = smd 0.5 x 1: 1 3.55,-7.34; 2 2.45,-7.34; 3 1.35,-7.34; 4 0.25,-7.34; 5 -0.85,-7.34; 6 -1.95,-7.34; 7 -3.05,-7.34; 8 -4.15,-7.34 | smd 0.72 x 0.78: 9 5.31,-4.66 | smd 1.05 x 1.08: 10 5.325,-3.39 | smd 1.05 x 1.2: 11 5.325,-0.78; 12 -5.325,-1.35 | smd 1.05 x 2.39: 13 -5.325,-4.535 | smd 2.91 x 0.55: 14 1.986,-0.105; 15 -2.204,-0.105
1X02 = drill 1.016 long: 1 -1.27,0; 2 1.27,0
BOURNS_SRP2010 = smd 0.559 x 1.6: P$1 -1.003,0; P$2 1.003,0
CONV_UWE1215S-3WR3 = drill 1 square: 1 -8.89,2.05 | drill 1: 2 -6.35,2.05; 3 -3.81,2.05; 5 1.27,2.05; 6 3.81,2.05; 7 6.35,2.05; 8 8.89,2.05
R0603 = smd 1 x 1.1: 1 -0.85,0; 2 0.85,0
B3F-10XX = drill 1.016 long: 1 -3.251,2.261; 2 3.251,2.261; 3 -3.251,-2.261; 4 3.251,-2.261
SOIC127P599X175-8N = smd 1.97 x 0.6: 1 -2.47,1.905; 2 -2.47,0.635; 3 -2.47,-0.635; 4 -2.47,-1.905; 5 2.47,-1.905; 6 2.47,-0.635; 7 2.47,0.635; 8 2.47,1.905
ES_DAISY_SEED_DOUBLE = drill 1.016 pad 1.88 square: 1 -7.493,24.13; B1 -10.033,24.13 | drill 1.016 pad 1.88: 2 -7.747,21.59; 3 -7.493,19.05; 4 -7.747,16.51; 5 -7.493,13.97; 6 -7.747,11.43; 7 -7.493,8.89; 8 -7.747,6.35; 9 -7.493,3.81; 10 -7.747,1.27; 11 -7.493,-1.27; 12 -7.747,-3.81; 13 -7.493,-6.35; 14 -7.747,-8.89; 15 -7.493,-11.43; 16 -7.747,-13.97; 17 -7.493,-16.51; 18 -7.747,-19.05; 19 -7.493,-21.59; 20 -7.747,-24.13; 21 7.493,-24.13; 22 7.747,-21.59; 23 7.493,-19.05; 24 7.747,-16.51; 25 7.493,-13.97; 26 7.747,-11.43; 27 7.493,-8.89; 28 7.747,-6.35; 29 7.493,-3.81; 30 7.747,-1.27; 31 7.493,1.27; 32 7.747,3.81; 33 7.493,6.35; 34 7.747,8.89; 35 7.493,11.43; 36 7.747,13.97; 37 7.493,16.51; 38 7.747,19.05; 39 7.493,21.59; 40 7.747,24.13; B2 -10.287,21.59; B3 -10.033,19.05; B4 -10.287,16.51; B5 -10.033,13.97; B6 -10.287,11.43; B7 -10.033,8.89; B8 -10.287,6.35; B9 -10.033,3.81; B10 -10.287,1.27; B11 -10.033,-1.27; B12 -10.287,-3.81; B13 -10.033,-6.35; B14 -10.287,-8.89; B15 -10.033,-11.43; B16 -10.287,-13.97; B17 -10.033,-16.51; B18 -10.287,-19.05; B19 -10.033,-21.59; B20 -10.287,-24.13; B21 10.033,-24.13; B22 10.287,-21.59; B23 10.033,-19.05; B24 10.287,-16.51; B25 10.033,-13.97; B26 10.287,-11.43; B27 10.033,-8.89; B28 10.287,-6.35; B29 10.033,-3.81; B30 10.287,-1.27; B31 10.033,1.27; B32 10.287,3.81; B33 10.033,6.35; B34 10.287,8.89; B35 10.033,11.43; B36 10.287,13.97; B37 10.033,16.51; B38 10.287,19.05; B39 10.033,21.59; B40 10.287,24.13
PAK100/2500-16 = drill 1 pad 1.422: 1 -8.89,-1.27; 2 -8.89,1.27; 3 -6.35,-1.27; 4 -6.35,1.27; 5 -3.81,-1.27; 6 -3.81,1.27; 7 -1.27,-1.27; 8 -1.27,1.27; 9 1.27,-1.27; 10 1.27,1.27; 11 3.81,-1.27; 12 3.81,1.27; 13 6.35,-1.27; 14 6.35,1.27; 15 8.89,-1.27; 16 8.89,1.27

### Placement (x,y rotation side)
C15  30.73,43.94 90 top
C16  23.62,51.05 270 top
C20  17.78,42.93 0 top
C21  44.45,16.51 270 top
C22  8.38,35.31 180 top
C23  25.91,35.05 0 top
C24  9.65,15.24 0 top
C25  44.7,43.43 270 top
C26  138.43,46.48 270 top
C27  137.92,18.03 270 top
C29  208.28,45.21 270 top
C30  18.8,39.88 270 top
C31  208.28,17.02 270 top
C32  20.07,35.05 0 top
J1  4.57,51.31 270 top
J2  109.73,37.59 180 top
JP12  9.65,50.8 270 top
L1  8.89,39.12 0 top
PS1  16.51,26.42 0 top
R1  44.7,39.12 270 top
R2  17.78,45.47 0 top
R3  17.53,51.56 180 top
R5  13.97,50.8 90 top
R6  40.64,13.97 180 top
R7  48.77,13.97 180 top
R8  44.45,11.94 270 top
R9  135.13,44.96 180 top
R12  142.49,44.96 180 top
R13  138.68,41.91 270 top
R14  134.11,16.51 180 top
R15  141.73,16.26 180 top
R16  137.92,13.46 270 top
R17  204.98,44.45 180 top
R18  212.34,44.45 180 top
R19  208.28,40.64 270 top
R20  204.72,15.24 180 top
R21  212.09,15.24 180 top
R22  208.28,12.19 270 top
R23  41.66,41.91 180 top
R24  59.94,54.61 270 top
R25  57.4,54.61 270 top
R27  65.02,43.69 270 top
R29  82.8,43.69 270 top
R30  85.34,43.69 270 top
R31  75.18,43.69 270 top
R32  72.64,43.69 270 top
R33  77.72,43.69 270 top
R34  80.26,43.69 270 top
R56  48.26,41.91 180 top
R93  80.26,54.61 90 top
R94  77.72,54.61 90 top
R95  75.18,54.61 90 top
R96  85.34,54.61 90 top
R97  82.8,54.61 90 top
S1  34.29,51.31 270 top
U1  25.15,42.42 180 top
U3  63.75,13.97 270 top
U4  157.23,42.67 270 top
U5  157.23,15.24 270 top
U6  227.33,42.42 270 top
U7  63.75,40.64 270 top
U8  227.33,14.22 270 top
X1  21.59,6.35 0 top

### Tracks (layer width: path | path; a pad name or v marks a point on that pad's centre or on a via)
+3V3  (via drill 0.35)
  Top 0.508: J2.4 109.47,53.34
  Top 0.61: R25.1 R24.1 R95.2 R94.2 R93.2 80.43,55.63 82.64,55.63 R97.2 R96.2 92.46,55.46 107.35,55.46 109.47,53.34 | U7.B38 U7.38 82.8,33.4 81.15,35.05 72.39,35.05 v70.61,36.83 | J2.4
  Top 1.016: 92.46,55.46 92.46,54.36 90.68,52.58 v90.68,44.45
  Bottom 1.016: v70.61,36.83 70.36,37.08 69.85,37.08 68.33,38.61 68.33,39.88 71.12,42.67 88.9,42.67 v90.68,44.45
+12V  (via drill 1)
  Top 0.61: U7.39 U7.B39 | U3.39 U3.B39 | U5.39 U5.B39 | U4.39 U4.B39 | U6.39 U6.B39 | U8.39 U8.B39
  Top 1.27: L1.P$1 5.08,39.12 3.05,37.08 3.05,18.8 6.6,15.24 C24.1 8.15,7.14 8.13,7.11 10.16,5.08 X1.1 X1.3 | v19.43,12.83 29.84,12.83 v29.97,12.95
  Bottom 1.27: X1.1 10.16,5.08 8.64,6.6 8.64,8.89 11.68,11.94 18.8,11.94 19.56,12.7 v19.43,12.83 | v29.97,12.95 37.08,20.07 37.08,26.16 v37.34,26.42
  pour Route15 (isolate 0.508): 1.78,20.83 27.94,20.83 37.13,11.64 250.65,11.64 254.97,15.95 254.97,25.61 38.66,25.61 38.66,21.64 38.1,21.08 36.32,22.86 36.32,34.29 37.85,35.81 112.52,35.81 112.82,35.51 262.33,35.51 264.16,33.69 264.16,3.3 262.84,1.98 0.56,1.98 0.51,2.03 0.51,19.56
+15V  (via drill 0.35)
  Top 0.61: U1.7 20.95,41.78 19.93,40.75 C30.1
  Top 1.016: v38.1,14.48 39.28,14.48 R6.2 | v131.07,16.52 131.08,16.51 R14.2 | v201.06,16.13 202.99,16.13 R20.2 | v38.86,41.91 R23.2 | v131.57,44.96 R9.2 | v202.18,42.93 203.71,44.45 R17.2 | C32.1 16.26,37.36 16.26,39.62 17.53,40.89 18.66,40.89 C30.1
  Top 1.27: C32.1 18.57,32.23 20.32,30.48 PS1.6
  Route15 1.016: PS1.6 20.32,27.45 24.65,23.12 24.77,23.25 24.91,23.11 29.46,23.11 32.38,20.19 | 32.38,20.19 36.58,16 | 36.58,16 v38.1,14.48 | 36.58,16 130.56,16 | 130.56,16 130.3,15.75 200.68,15.75 v201.06,16.13 | 130.56,16 v131.07,16.52 | 32.38,20.19 32.51,20.32 32.51,35.56 38.23,41.27 | 38.23,41.27 v38.86,41.91 | 38.23,41.27 56.52,41.27 57.91,42.67 87.38,42.67 89.6,40.45 96.54,40.45 99.14,37.85 124.21,37.85 127.38,41.02 | v131.57,44.96 131.32,44.96 127.38,41.02 | 127.38,41.02 129.03,39.37 199.14,39.37 202.18,42.42 v202.18,42.93
  pour Route15 (isolate 0.508): 0.76,56.64 0.76,22.61 28.7,22.61 33.78,17.53 34.54,17.53 34.54,38.1 41.15,38.1 41.4,37.85 41.4,55.88 1.52,55.88
-15V  (via drill 0.35)
  Top 0.61: C15.2 28.11,44.82 U1.4
  Top 0.813: C15.2 33.27,44.82 33.53,44.56 38.49,44.56 38.61,44.45 v38.35,44.45
  Top 1.016: v50.67,43.56 49.11,42 R56.1 | v145.16,46.1 144.02,44.96 R12.1 | v215.39,45.47 214.21,45.47 R18.1 | PS1.8 28.72,25.15 32,25.15 v33.78,23.37 | v51.05,17.78 51.05,15.41 R7.1 | v145.03,18.54 144.87,18.54 R15.1 | v215.39,16.76 213.87,15.24 R21.1
  Top 1.27: C23.2 27.41,30.47 PS1.8
  Route15 1.016: PS1.8 30.23,33.29 30.23,37.85 36.83,44.45 v38.35,44.45 49.53,44.45 | 49.53,44.45 50.55,43.43 v50.67,43.56 | 49.53,44.45 50.04,44.96 89.15,44.96 90.17,45.97 94.49,45.97 100.84,39.62 123.19,39.62 130.56,46.99 144.53,46.99 145.29,46.23 v145.16,46.1 145.54,45.72 197.53,45.72 199.2,47.2 213.68,47.18 v215.39,45.47 | v33.78,23.37 39.37,17.78 v51.05,17.78 129.29,17.78 130.56,19.05 145.03,19.05 145.29,18.8 | 145.29,18.8 v145.03,18.54 | 145.29,18.8 213.87,18.8 215.65,17.02 v215.39,16.76
CLK  (via drill 0.35)
  Top 0.508: 110.58,51.22 J2.5 | R32.2 v72.64,40.13
  Top 0.61: v110.49,51.31 110.58,51.22
  Bottom 0.508: v72.64,40.13 73.66,40.13 73.91,39.88 91.44,39.88 93.22,41.66 96.52,41.66 101.6,46.74 106.17,46.74 110.49,51.05
  Bottom 0.61: 110.49,51.05 v110.49,51.31
CMD  (via drill 0.35)
  Top 0.508: v107.7,52.07 108.46,51.31 108.46,45.01 | R31.2 v75.18,41.15
  Top 0.61: J2.3 108.46,45.01
  Bottom 0.508: v75.18,41.15 90.93,41.15 92.71,42.93 96.01,42.93 101.09,48.01 105.41,48.01 107.7,50.29 v107.7,52.07
DAT0
  Top 0.508: R33.2 82.72,37.85 90.17,37.85 92.34,35.67 92.34,35.62 93.79,34.18 96.71,34.18 97.33,34.8 115.57,34.8 117.86,37.08 117.86,46.23 116.2,47.88 114.17,47.88 112.78,46.48 J2.7
DAT1
  Top 0.508: R34.2 83.48,39.62 91.14,39.62 92.01,40.5 97.68,40.5 102.11,36.07 114.81,36.07 116.59,37.85 116.59,45.72 115.82,46.49 114.63,46.5 113.88,45.75 J2.8
DAT2
  Top 0.508: R29.2 82.8,42.33 83.48,41.66 83.57,41.66 84.07,41.15 90.17,41.15 90.93,41.91 96.01,41.91 103.24,49.14 105.04,49.14 106.17,48.01 106.18,47.73 J2.1
DAT3
  Top 0.508: R30.2 88.14,42.84 88.39,43.09 95.67,43.09 102.62,50.04 105.66,50.04 107.28,48.42 J2.2
DGND4  (via drill 0.35)
  Top 0.305: v115.57,44.96 115.57,44.2 115.05,43.68 J2.13 | v102.62,41.15 102.62,40.16 J2.11
  Top 0.508: J2.10 J2.11 | J2.12 J2.13 | J2.6 111.68,50.46 112.78,51.56 v113.54,51.56
  Top 0.61: U7.35 U7.B35 | U7.36 U7.B36 | U7.37 U7.B37 | U7.40 U7.B40 | U3.37 U3.B37 | U3.36 U3.B36 | U4.37 U4.B37 | U6.B20 U6.20 | U6.36 U6.B36 | U6.35 U6.B35 | U8.B20 U8.20 | S1.3 S1.4 32.03,47.73 34.04,45.72 38.86,45.72 39.62,46.48 U7.20
  Top 1.27: C22.2 6.88,29.2 PS1.1 | C24.2 12.7,13.69 X1.2 X1.4
  pour Route2 (isolate 0.508): 1.52,26.42 1.52,38.61 3.56,40.64 14.22,40.64 14.99,39.88 14.99,28.96 17.53,26.42 25.4,26.42 36.83,37.85 36.83,51.05 42.93,57.15 261.87,57.15 264.41,54.61 264.41,3.3 262.89,1.78 0.25,1.78 0.25,25.15
GNDINT  (via drill 0.35)
  Top 0.61: U1.3 27.63,43.07 C15.1 | R5.1 10.07,49.95 JP12.2 4.84,49.53 4.57,49.8 J1.3 J1.4
  Top 1.016: C30.2 19.16,39 21.59,36.58 21.59,35.08 C32.2 | C15.1 31.89,43.07 32,43.18 v32.77,43.18
  Top 1.27: C32.2 21.57,33.3 22.86,32 | 22.86,32 PS1.7 | C23.1 24.41,33.55 22.86,32
  pour Route2 (isolate 0.508): 18.03,27.18 25.15,27.18 36.07,38.1 36.07,50.8 35.81,51.05 41.15,56.39 41.15,56.64 0.76,56.64 0.51,56.39 0.51,43.69 2.29,41.91 15.49,41.91 16,41.4 16,29.21
I2C_SCL  (via drill 0.35)
  Top 0.305: v186.69,8.89 183.39,12.19 162.81,12.19 162.56,11.94 153.42,21.08 U5.12 | U5.B12 153.42,27.43 152.4,28.45 104.14,28.45 95.5,19.81 61.21,19.81 59.94,21.08 U3.12 | U7.12 59.94,43.18 51.56,34.8 39.12,34.8 38.1,33.78 38.1,29.72 39.12,28.7 56.9,28.7 59.94,25.65 U3.B12
  Top 0.61: R24.2 U7.B12 U7.12 | U3.B12 U3.12 | U5.B12 U5.12 | U4.B12 U4.12 | U6.B12 U6.12 | U8.B12 U8.12
  Bottom 0.305: U6.12 223.52,40.39 219.38,36.25 202.65,36.25 201.21,34.8 201.17,34.8 201.17,27.43 202.44,26.16 222.25,26.16 223.52,24.89 U8.B12 | U8.12 223.52,13.21 219.2,8.89 v186.69,8.89 | U4.12 153.42,40.89 149.28,36.75 132.04,36.75 131.27,35.98 131.27,31.04 134.62,27.69 152.4,27.69 153.42,26.67 U5.B12
I2C_SDA  (via drill 0.35)
  Top 0.305: v155.96,20.83 155.96,20.32 162.81,13.46 184.4,13.46 v186.9,10.97 | U5.B13 150.62,25.53 150.62,26.67 150.11,27.18 105.41,27.18 96.77,18.54 59.18,18.54 57.4,20.32 U3.13 | U7.13 57.4,42.67 50.29,35.56 38.86,35.56 37.34,34.04 37.34,29.21 38.61,27.94 54.61,27.94 57.4,25.15 U3.B13
  Top 0.61: R25.2 U7.B13 U7.13 | U3.B13 U3.13 | U5.B13 U5.13 | U4.B13 U4.13 | U6.B13 U6.13
  Bottom 0.305: U6.13 220.98,39.12 218.95,37.08 202.18,37.08 200.15,35.05 200.15,21.34 201.68,19.81 219.07,19.81 U8.13 220.98,12.45 218.23,9.7 188.17,9.7 v186.9,10.97 | v155.96,20.83 151.38,20.83 150.62,21.59 150.62,22.48 U5.13 | U4.13 150.88,40.39 148.08,37.59 131.83,37.59 130.3,36.07 130.3,30.73 134.11,26.92 150.11,26.92 150.88,26.16 U5.B13
  Bottom 0.813: U8.B13 U8.13
MASTER_SIGNAL  (via drill 0.35)
  Top 0.406: v122.68,52.07 127.51,52.07 130.56,55.12 180.34,55.12 181.36,54.1 U4.B1 | U4.B1 U4.1 | U4.B1 181.36,53.85 182.37,54.86 250.44,54.86 251.46,53.85 U6.B1 U6.1 257.3,44.07 257.3,27.94 253.62,24.26 U8.B1 U8.1 240.28,10.54 240.28,10.16 239.52,9.4 191.01,9.4 183.39,17.02 175.77,17.02 v175.77,17.12 | v93.47,21.59 88.01,21.59 | 88.01,21.59 U3.1 | U3.B1 87.88,21.72 88.01,21.59 | U5.B1 U5.1
  Bottom 0.406: U7.B1 U7.1 89.79,46.23 96.77,46.23 100.58,50.04 104.65,50.04 105.41,50.8 105.41,52.07 106.68,53.34 121.67,53.34 122.68,52.32 v122.68,52.07 | U5.1 181.36,22.7 v175.77,17.12 149.96,17.12 145.03,12.19 142.24,12.19 141.22,11.18 141.22,10.92 105.66,10.92 95,21.59 v93.47,21.59
MISO_2
  Top 0.61: R27.1 U7.10 U7.B10
MISO_2_P1
  Top 0.61: U3.B10 U3.10
MISO_2_P2
  Top 0.61: U4.B10 U4.10
MISO_2_P3
  Top 0.61: U5.B10 U5.10
MISO_2_P4
  Top 0.254: U6.B10 U6.10
MISO_2_P5
  Top 0.254: U8.B10 U8.10
MONO_OUTPUT
  Top 0.61: 18.76,43.05 18.63,43.18 R2.2 21.82,48.65 | U1.6 18.76,43.05 | 18.76,43.05 C20.2
  Top 0.813: C16.+ 21.82,48.65
MOSI_2  (via drill 0.35)
  Top 0.254: U6.B11 U6.11 236.85,39.12 250.44,39.12 253.75,35.81 253.75,31.24 252.98,30.48 232.28,30.48 U8.B11 U8.11
  Top 0.305: U5.B11 160.91,30.23 182.12,30.23 183.64,31.75 183.67,36.6 178.56,41.91 164.21,41.91 156.02,50.1 U4.11 155.96,44.2 149.86,38.1 123.45,38.1 118.84,33.49 98.26,33.49 90.42,25.65 v71.37,25.65 | U8.B11 226.06,25.15 224.79,26.42 192.53,26.42 184.91,18.8 159.89,18.8 U5.11 | U7.11 62.48,38.86 v63.5,37.85
  Top 0.61: U7.B11 U7.11 | U3.B11 U3.11 | U5.B11 U5.11 | U4.B11 156.02,52.64 156.02,50.1
  Bottom 0.305: X1.12 27.18,9.4 57.91,9.4 62.48,13.97 U3.11 | v63.5,37.85 61.47,35.81 52.58,35.81 52.07,35.31 38.61,35.31 37.08,33.78 37.08,29.97 38.86,28.19 59.94,28.19 62.48,25.65 62.48,24.89 | 62.48,24.89 62.48,23.37 | v71.37,25.65 63.25,25.65 62.48,24.89
  Bottom 0.61: U3.B11 62.48,23.37 U3.11
N$1
  Top 0.61: U5.31 U5.B31
N$2
  Top 0.305: C21.2 45.49,13.97
  Top 0.61: R8.1 C21.2 43.41,13.97 R6.1 | 45.49,13.97 R7.2
N$3
  Top 0.61: U6.31 U6.B31
N$4  (via drill 0.35)
  Top 0.61: R1.2 35.39,38.27 35.39,38.01 | U1.2 31.62,41.78 v34.04,39.37 35.39,38.01 | R8.2 38.19,11.09 35.39,13.88 35.39,38.01 | R19.2 208.11,39.62 v206.25,39.62 | R22.2 201.76,11.34 200.66,12.45 v200.15,12.45 | R16.2 134.28,12.61 134.11,12.45 v133.86,12.45 | R13.2 131.41,41.06 v131.06,41.4
  Top 0.813: R2.1 16.93,44.2 | 16.93,44.2 C20.1 | v15.49,44.2 16.93,44.2
  Bottom 0.61: v206.25,39.62 205.49,39.62 204.47,40.64 201.93,40.64 197.61,44.96 | 126.75,55.12 194.82,55.12 197.61,52.32 197.61,44.96 | 126.75,55.12 40.39,55.12 34.29,49.02 34.29,45.97 34.29,39.62 v34.04,39.37 | v200.15,12.45 197.61,14.99 197.61,44.96 | v133.86,12.45 130.81,12.45 126.75,16.51 126.75,45.72 | 126.75,45.72 126.75,55.12 | v131.06,41.4 126.75,45.72
  Bottom 0.813: 34.29,45.97 34.04,45.72 16.26,45.72 15.24,44.7 15.24,44.2 v15.49,44.2
N$5
  Top 0.61: R3.1 20.27,53.45 C16.-
N$6
  Top 0.61: R3.2 14.06,51.56 R5.2 10.07,51.65 JP12.1 4.81,52.07 J1.2 J1.1
N$7
  Top 0.61: C25.2 R1.1 | C25.2 44.73,41.91 R56.2 | C25.2 44.68,41.91 R23.1
N$8
  Top 0.61: C26.2 138.68,44.73 R13.1
  Top 0.813: C26.2 138.41,44.96
  Top 1.016: 138.41,44.96 R9.1 | C26.2 141.62,44.98 R12.2
N$9
  Top 0.61: C27.2 R16.1 | C27.2 138.2,16.26 R15.2 | C27.2 137.9,16.51 R14.1
N$10
  Top 0.61: C29.2 208.3,43.69 210.73,43.69 R18.2 | C29.2 206.57,43.71 R17.1 | C29.2 R19.1
N$11
  Top 0.61: C31.2 R22.1
  Top 1.016: R20.1 208,15.24 C31.2 210.96,15.52 R21.2
N$12
  Top 0.61: U7.B19 U7.19
N$13
  Top 0.61: U7.B17 U7.17
N$14
  Top 0.61: U7.B16 U7.16
N$15
  Top 0.61: U7.B15 U7.15
N$17
  Top 0.61: U8.31 U8.B31
N$18
  Top 0.61: U8.26 U8.B26
N$19
  Top 0.61: U6.26 U6.B26
N$20
  Top 0.61: U7.34 U7.B34
N$21
  Top 0.61: U7.33 U7.B33
N$22
  Top 0.61: U7.32 U7.B32
N$23
  Top 0.61: U5.26 U5.B26
N$24  (via drill 0.35)
  Top 0.305: R27.2 65.02,41.4 64.77,41.15 v64.52,41.15
  Bottom 0.305: v64.52,41.15 60.2,36.83 52.32,36.83 51.56,36.07 38.1,36.07 30.73,28.7 30.73,16.76 24.13,10.16 24.13,6.35 X1.11
N$25
  Top 0.61: U7.28 U7.B28
N$26
  Top 0.61: U7.27 U7.B27
N$27
  Top 0.61: U4.26 U4.B26
N$28
  Top 0.61: U3.26 U3.B26
N$29
  Top 0.61: U3.21 U3.B21
N$30
  Top 0.61: U7.24 U7.B24
N$31
  Top 0.61: U7.23 U7.B23
N$32
  Top 0.61: U7.22 U7.B22
N$33
  Top 0.305: U3.B19 U3.19
N$34
  Top 0.61: U3.B17 U3.17
N$35
  Top 0.61: U3.B16 U3.16
N$36
  Top 0.61: U3.B15 U3.15
N$37
  Top 0.61: U3.B14 U3.14
N$38
  Top 0.61: U7.26 U7.B26
N$39
  Top 0.61: U3.38 U3.B38 | U3.35 U3.B35
  Top 0.813: U3.38 82.8,7.37 81.79,8.38 76.2,8.38 75.18,7.37 U3.35
N$40
  Top 0.61: U3.34 U3.B34
N$41
  Top 0.61: U3.33 U3.B33
N$42
  Top 0.61: U3.32 U3.B32
N$43
  Top 0.61: U3.28 U3.B28
N$44
  Top 0.61: U3.27 U3.B27
N$45
  Top 0.61: U7.21 U7.B21
N$46
  Top 0.61: U3.24 U3.B24
N$47
  Top 0.61: U3.23 U3.B23
N$48
  Top 0.61: U3.22 U3.B22
N$49
  Top 0.61: U4.21 U4.B21
N$50
  Top 0.61: U4.B19 U4.19
N$51
  Top 0.61: U4.B17 U4.17
N$52
  Top 0.61: U4.B16 U4.16
N$53
  Top 0.61: U4.B15 U4.15
N$54
  Top 0.61: U4.B14 U4.14
N$55
  Top 0.61: U7.B14 U7.14 | S1.1 S1.2
  Bottom 0.61: S1.2 36.58,48.03 36.58,46.74 37.34,45.97 54.1,45.97 54.86,46.74 U7.14
N$56
  Top 0.406: U3.B2 U3.2
N$57
  Top 0.61: U4.34 U4.B34
N$58
  Top 0.61: U4.33 U4.B33
N$59
  Top 0.61: U4.32 U4.B32
N$60
  Top 0.61: U4.28 U4.B28
N$61
  Top 0.61: U4.27 U4.B27
N$62
  Top 0.61: U4.24 U4.B24
N$63
  Top 0.61: U4.23 U4.B23
N$64
  Top 0.61: U4.22 U4.B22
N$65
  Top 0.61: U5.21 U5.B21
N$66
  Top 0.61: U5.B19 U5.19
N$67
  Top 0.61: U5.B17 U5.17
N$68
  Top 0.61: U5.B16 U5.16
N$69
  Top 0.61: U5.B15 U5.15
N$70
  Top 0.61: U5.B14 U5.14
N$71
  Top 0.406: U3.B3 U3.3
N$72
  Top 0.406: U3.B4 U3.4
N$73
  Top 0.61: U5.34 U5.B34
N$74
  Top 0.61: U5.33 U5.B33
N$75
  Top 0.61: U5.32 U5.B32
N$76
  Top 0.61: U5.28 U5.B28
N$77
  Top 0.61: U5.27 U5.B27
N$78
  Top 0.61: U5.24 U5.B24
N$79
  Top 0.61: U5.23 U5.B23
N$80
  Top 0.61: U5.22 U5.B22
N$81
  Top 0.61: L1.P$2 9.89,35.32 C22.1
  Top 1.27: C22.1 9.88,28.74 PS1.2
N$82
  Top 0.61: U6.21 U6.B21
N$83
  Top 0.61: U6.B19 U6.19
N$84
  Top 0.61: U6.B17 U6.17
N$85
  Top 0.61: U6.B16 U6.16
N$86
  Top 0.61: U6.B15 U6.15
N$87
  Top 0.61: U6.B14 U6.14
N$88
  Top 0.61: U6.B38 U6.38 244.09,34.67 U6.37 U6.B37
N$89
  Top 0.406: U3.B5 U3.5
N$90
  Top 0.61: U6.34 U6.B34
N$91
  Top 0.61: U6.33 U6.B33
N$92
  Top 0.61: U6.32 U6.B32
N$93
  Top 0.61: U6.28 U6.B28
N$94
  Top 0.61: U6.27 U6.B27
N$95
  Top 0.61: U6.24 U6.B24
N$96
  Top 0.61: U6.23 U6.B23
N$97
  Top 0.61: U6.22 U6.B22
N$98
  Top 0.61: U8.21 U8.B21
N$99
  Top 0.61: U8.B19 U8.19
N$100
  Top 0.61: U8.B17 U8.17
N$101
  Top 0.61: U8.B16 U8.16
N$102
  Top 0.61: U8.B15 U8.15
N$103
  Top 0.61: U8.B14 U8.14
N$104
  Top 0.61: U8.B38 U8.38 246.38,7.37 245.36,8.38 243.84,8.38 | U8.B37 U8.37 243.84,8.38 | U8.B35 U8.35 240.03,8 240.03,8.38 243.84,8.38
N$105
  Top 0.406: U3.B6 U3.6
N$106
  Top 0.406: U3.B7 U3.7
N$108
  Top 0.61: U8.34 U8.B34
N$109
  Top 0.61: U8.33 U8.B33
N$110
  Top 0.61: U8.32 U8.B32
N$111
  Top 0.61: U8.28 U8.B28
N$112
  Top 0.61: U8.27 U8.B27
N$113
  Top 0.61: U8.24 U8.B24
N$114
  Top 0.61: U8.23 U8.B23
N$115
  Top 0.61: U8.22 205.74,4.57 205.99,4.32 205.99,4.19 U8.B22
N$116
  Top 0.406: U4.B2 U4.2
N$117
  Top 0.406: U4.B3 U4.3
N$118
  Top 0.406: U4.B4 U4.4
N$119
  Top 0.406: U4.B5 U4.5
N$120
  Top 0.406: U4.B6 U4.6
N$121
  Top 0.406: U4.B7 U4.7
N$123
  Top 0.406: U5.B2 U5.2
N$124
  Top 0.406: U5.B3 U5.3
N$125
  Top 0.406: U5.B4 U5.4
N$126
  Top 0.406: U5.B5 U5.5
N$127
  Top 0.406: U5.B6 U5.6
N$128
  Top 0.406: U5.B7 U5.7
N$130
  Top 0.406: U6.B2 U6.2
N$131
  Top 0.406: U6.B3 U6.3
N$132
  Top 0.406: U6.B4 U6.4
N$133
  Top 0.406: U6.B5 U6.5
N$134
  Top 0.406: U6.B6 U6.6
N$135
  Top 0.406: U6.B7 U6.7
N$136
  Top 0.406: U8.B2 U8.2
N$137
  Top 0.406: U8.B3 U8.3
N$138
  Top 0.406: U8.B4 U8.4
N$139
  Top 0.406: U8.B5 U8.5
N$140
  Bottom 0.406: U8.B6 U8.6
N$141
  Bottom 0.406: U8.B7 U8.7
OUT1
  Top 0.61: 44.7,47.75 C25.1 | U7.18 U7.B18
  Top 0.813: U7.18 44.7,47.75
OUT2
  Top 0.305: U3.18 U3.B18
  Top 0.61: U3.18 44.7,18.26 C21.1
OUT3
  Top 0.61: C26.1 138.43,50.16 U4.18 U4.B18
OUT4
  Top 0.61: C27.1 138.18,19.79 U5.18 U5.B18
OUT5
  Top 0.61: C29.1 U6.18 U6.B18
OUT6
  Top 0.61: C31.1 U8.18 U8.B18
PA1_SD_DETECT  (via drill 0.35)
  Top 0.305: v67.31,10.41 65.02,8.12 U3.31
  Top 0.508: 65.02,33.78 69.98,38.73 v70.23,38.73 | 104.05,42.25 103.38,42.93 v102.11,42.93
  Top 0.61: 65.02,33.78 U7.31 U7.B31 | J2.9 104.05,42.25 | U3.31 U3.B31
  Bottom 0.305: U7.B31 67.69,27.94 90.93,27.94 92.2,26.67 92.2,19.56 84.07,11.43 72.64,11.43 71.63,10.41 v67.31,10.41
  Bottom 0.508: v70.23,38.73 72.01,38.73 72.14,38.61 92.15,38.61 94.05,40.5 99.94,40.5 102.11,42.67 v102.11,42.93
PA1_SD_DETECT1
  Top 0.61: U4.31 U4.B31
PULLUPED
  Top 0.61: U5.38 U5.B38 174.62,3.3 172.85,3.3 U5.B36 | U5.36 U5.B36 | U5.35 U5.B35 168.91,4.95 U5.B36
PULLUPED2
  Top 0.61: U4.B38 U4.38 176.28,36.58 175.77,37.08 172.21,37.08 171.2,36.07 U4.36 U4.B36
SCLK_2  (via drill 0.35)
  Top 0.254: U8.9 U8.B9 231.14,26.67 234.19,29.72 253.49,29.72 254.76,30.99 254.76,36.58 250.95,40.39 238.25,40.39 231.14,47.5 U6.9 U6.B9
  Top 0.305: U4.9 161.04,49.53 167.13,43.43 178.82,43.43 185.3,36.96 185.42,31.5 182.88,28.96 163.32,28.96 161.04,26.67 U5.B9 | U5.9 163.96,19.81 183.39,19.81 190.75,27.18 v216.41,27.18 | U7.9 69.6,46.1 69.6,40.64 74.17,36.07 87.12,36.07 90.17,33.02 v90.17,30.73 90.17,30.48 87.88,28.19 69.34,28.19 67.56,26.42 U3.B9 | v158.5,41.4 154.43,37.34 123.95,37.34 118.36,31.75 98.81,31.75 94.49,27.43 v94.36,27.56
  Top 0.61: U7.B9 U7.9 | U3.B9 U3.9 | U5.B9 U5.9 | U4.B9 U4.9
  Bottom 0.305: X1.10 22.86,10.41 29.72,17.27 29.72,29.21 37.34,36.83 50.59,36.83 51.79,38.02 59.61,38.02 67.56,45.97 U7.9 | v216.41,27.18 224.45,27.18 225.47,26.16 230.38,26.16 231.14,25.4 U8.B9 | U4.9 161.04,43.94 v158.5,41.4 | v94.36,27.56 93.34,27.56 v90.17,30.73
SD_CLK
  Top 0.61: R32.1 U7.7 U7.B7
SD_CMD
  Top 0.305: U7.B6 U7.6
  Top 0.61: R31.1 U7.6 R95.1
SD_DAT0
  Top 0.61: R33.1 U7.5 U7.B5 R94.1
SD_DAT1
  Top 0.61: R34.1 U7.4 U7.B4 R93.1
SD_DAT2
  Top 0.61: R29.1 U7.3 U7.B3 R97.1
SD_DAT3
  Top 0.61: R30.1 U7.2 U7.B2 R96.1
SPI6_CLK
  Top 0.305: U8.B29 221.36,2.03 155.7,2.03 153.67,4.06 153.67,4.95 U5.B29 153.42,5.08 153.42,4.32 151.89,2.79 150.37,2.79 149.86,2.29 131.32,2.29 122.17,11.43 64.26,11.43 59.94,7.11 U3.29
  Top 0.61: U7.29 U7.B29 | U3.29 U3.B29 | U5.29 153.42,5.08 | U4.29 U4.B29 | U6.29 U6.B29
  Top 0.813: U8.29 U8.B29
  Bottom 0.254: U8.B29 223.52,7.37 228.09,11.94 252.48,11.94 255.02,14.48 255.02,25.4 252.98,27.43 227.08,27.43 223.52,30.99 U6.B29
  Bottom 0.305: X1.6 17.78,7.37 16.51,6.1 16.51,3.56 18.54,1.52 57.53,1.52 U3.B29 | U5.29 153.42,8.38 158.75,13.72 177.55,13.72 184.38,20.55 184.38,27.2 182.88,28.7 155.96,28.7 153.42,31.24 U4.B29 | U7.B29 60.96,29.59 60.96,28.45 62.99,26.42 89.15,26.42 90.17,25.4 90.17,20.57 83.82,14.22 67.31,14.22 59.94,6.86 U3.29
SPI6_MOSI  (via drill 0.35)
  Top 0.305: U3.25 49.78,7.87 54.1,12.19 120.65,12.19 | U5.25 141.48,9.53 125.73,9.53 123.06,12.19 120.65,12.19 | 120.65,12.19 107.19,25.65 106.43,25.65 v106.43,25.91
  Top 0.61: U7.25 U7.B25 | U5.25 U5.B25 | U4.25 U4.B25
  Top 0.813: U3.25 U3.B25
  Bottom 0.254: U8.B25 U8.25 214.88,8.26 223.01,8.26 227.71,12.95 251.46,12.95 254,15.49 254,25.15 252.22,26.92 226.19,26.92 223.01,30.1 215.65,30.1 U6.B25 U6.25
  Bottom 0.305: U3.B25 48.13,2.29 22.86,2.29 21.65,3.5 21.65,6.54 20.57,7.62 X1.8 | U5.25 150.75,15.24 177.29,15.24 183.39,21.34 183.39,26.67 182.37,27.69 155.32,27.69 152.4,30.61 145.29,30.61 U4.B25 | U8.B25 213.36,3.3 212.09,2.03 144.78,2.03 143.26,3.56 U5.B25 | v106.43,25.91 103.38,28.96 96.01,28.96 90.17,34.8 53.12,34.8 52.74,34.42 51.05,34.42 U7.25
SPI6_NSS  (via drill 0.35)
  Top 0.254: U8.B30 U8.30
  Top 0.305: v58.93,39.88 62.48,36.32 U7.30 | U8.30 226.06,6.6 224.54,8.13 189.99,8.13 189.23,7.37 185.93,7.37 182.88,10.41 157.73,10.41 156.34,9.02 | U5.30 155.96,8.64 156.34,9.02 | v143.26,10.67 143.76,10.16 155.19,10.16 156.34,9.02
  Top 0.61: U7.30 U7.B30 | U3.30 U3.B30 | U4.30 U4.B30 | U6.30 U6.B30
  Bottom 0.254: U8.30 226.06,7.62 229.36,10.92 252.98,10.92 256.03,13.97 256.03,25.65 253.75,27.94 229.87,27.94 226.06,31.75 U6.B30
  Bottom 0.305: X1.5 19.05,6.35 19.05,8.64 28.45,18.03 28.45,29.21 36.83,37.59 49.78,37.59 51.31,39.12 58.17,39.12 v58.93,39.88 | U5.B30 U5.30 155.96,9.65 158.5,12.19 178.05,12.19 185.67,19.81 185.67,27.43 183.39,29.72 157.48,29.72 155.96,31.24 U4.B30 | 64.01,9.4 141.99,9.4 v143.26,10.67 | 64.01,9.4 62.48,7.87 U3.30 | U7.B30 62.23,30.1 62.23,28.45 63.5,27.18 90.42,27.18 91.19,26.42 91.19,19.81 84.59,13.21 67.82,13.21 64.01,9.4
SS_2  (via drill 0.35)
  Top 0.254: U6.8 233.68,47.24 239.27,41.66 251.46,41.66 255.78,37.34 255.78,30.73 254,28.96 v235.2,28.96 233.68,27.43 U8.B8 U8.8
  Top 0.305: U6.B8 U6.8 | U4.8 163.58,49.53 167.39,45.72 178.31,45.72 186.73,37.38 186.71,30.5 183.9,27.69 165.1,27.69 163.58,26.16 163.58,23.11 U5.8 165.74,20.83 182.12,20.83 189.23,27.94 227.84,27.94 v229.62,29.72 | U7.8 70.61,47.88 70.61,40.64 74.42,36.83 87.88,36.83 91.44,33.27 v91.44,31.5 91.44,29.97 88.9,27.43 71.37,27.43 70.1,26.16 U3.B8 | v135.64,29.72 99.82,29.72 v97.79,27.69
  Top 0.61: U7.B8 U7.8 | U3.B8 U3.8
  Top 0.813: U5.B8 163.58,23.11
  Bottom 0.305: X1.9 24.64,3.3 33.27,3.3 38.28,8.31 58.77,8.31 63.58,13.12 63.58,14.43 70.1,20.95 | v235.2,28.96 234.7,28.96 233.93,29.72 v229.62,29.72 | U5.B8 162.18,26.92 154.69,26.92 151.89,29.72 v135.64,29.72 | v97.79,27.69 95.76,27.69 92.2,31.24 91.44,31.24 v91.44,31.5
  Bottom 0.61: 70.1,20.95 U3.8 | U4.B8 U4.8

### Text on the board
tPlace: G | H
